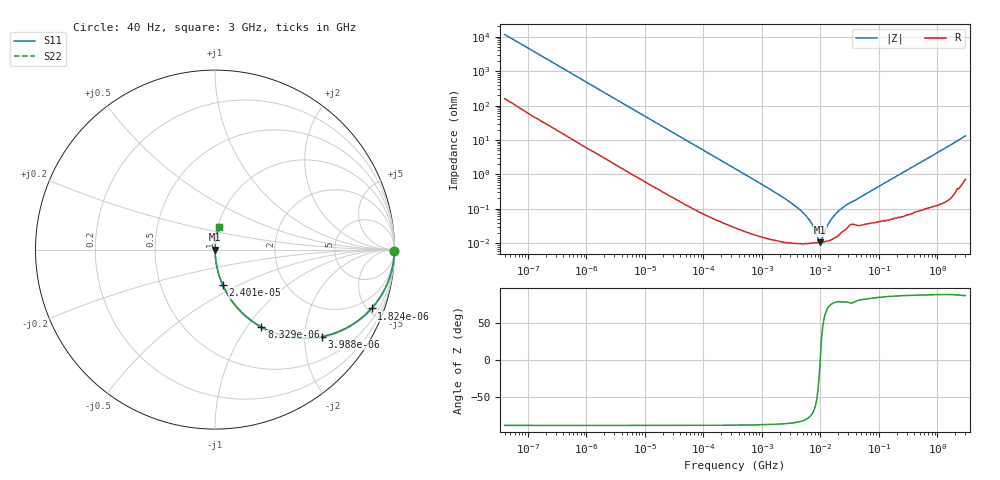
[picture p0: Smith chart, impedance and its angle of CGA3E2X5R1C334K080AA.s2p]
! S-parameter Generated by TDK Corporation
! Copyright(C) 2015 TDK Corporation.
! All Rights Reserved.
! TDK P/N: CGA3E2X5R1C334K080AA (Multilayer Ceramic Chip Capacitors)
! Property: C=330nF
! Size(LxWxT): 1.6x0.8x0.8mm, 0.063x0.031x0.031inches
! Model Type: s2p (Touchstone File Format Version 1.0)
! Frequency: DC=Yes Start=0.00004MHz Stop=3000MHz 396points Log-sweep
! Note: This model was converted from impedance.
! Model Generated on Jun. 23, 2015
! Hash(MD5):
! Port Assignments:
!  1 ---| |--- 2
! Applicable Conditions:
!  Temperature = 25 degC
!  DC Bias Voltage = 0 V
!  Small Signal Operation
! Terms and conditions regarding TDK Simulation Models
! (1)This simulation model is being provided solely for informational purposes. Please refer to the specifications of the products in terms of detailed characteristics of such products.
! (2)In no event shall TDK Corporation of any of its subsidiaries be liable for any loss or damage arising, directly or indirectly,
!  From any information contained in this simulation model, including, but not limited to loss or damages arising from any inaccuracies, omissions or errors in connection with such information.
! (3)Any and all copyrights on this simulation model are owned by TDK Corporation.
!  Duplication or redistribution of this simulation model without prior written permission from TDK Corporation is prohibited.
! (4)This simulation model is subject to any modification or change without any prior notice.
! (5)Neither TDK Corporation nor any of its subsidiaries shall make any warranty, express or implied,
!  Including but not limited to the correctness, implied warranties of merchantability and fitness for a particular purpose with respect to this simulation models.
! (6)The use of this simulation model shall be deemed to have consented to the terms and conditions hereof.
# MHz S MA R 50
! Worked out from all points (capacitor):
!   395 points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, 40 Hz to 3 GHz, reference 50 ohm
!   read as one part in series: C = 340 nF near 41.88 Hz
!   lowest |Z| = 10.7 mohm at 9.97 MHz (marker M1)
!   series resonance near 9.89 MHz, so ESL is about 760 pH
!   S11 on the Smith chart (normalised r, x): 40 Hz: open; 1.824 kHz: 1.07, -5.30; 3.988 kHz: 1.03, -2.44; 8.329 kHz: 1.01, -1.17; 24.01 kHz: 1.01, -0.41; 3 GHz: 1.01, +0.26
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4e-05  0.9998 -0.5  0.008564 88.7  0.008564 88.7  0.9998 -0.5
0.0002520917  0.9979 -3.0  0.05281 86.2  0.05281 86.2  0.9979 -3.0
0.000834128  0.9832 -9.8  0.1707 79.5  0.1707 79.5  0.9832 -9.8
0.001823978  0.9317 -20.6  0.3517 68.7  0.3517 68.7  0.9317 -20.6
0.003988472  0.7684 -39.1  0.6306 50.2  0.6306 50.2  0.7684 -39.1
0.008329251  0.5036 -59.0  0.8577 30.2  0.8577 30.2  0.5036 -59.0
0.01739424  0.2716 -73.5  0.959 15.8  0.959 15.8  0.2716 -73.5
0.02400588  0.2014 -77.7  0.977 11.6  0.977 11.6  0.2014 -77.7
0.0724464  0.06922 -85.3  0.9967 4.0  0.9967 4.0  0.06922 -85.3
0.3464102  0.01478 -88.1  0.9996 0.8  0.9996 0.8  0.01478 -88.1
3.154924  0.00149 -86.0  0.9999 0.1  0.9999 0.1  0.00149 -86.0
4.998775  0.0007861 -83.0  0.9999 0.0  0.9999 0.0  0.0007861 -83.0
7.22376  0.000355 -73.4  0.9999 0.0  0.9999 0.0  0.000355 -73.4
9.521122  0.0001138 -21.5  0.9999 0.0  0.9999 0.0  0.0001138 -21.5
9.969551  0.0001069 4.8  0.9999 -0.0  0.9999 -0.0  0.0001069 4.8
12.54911  0.0002763 65.6  0.9999 -0.0  0.9999 -0.0  0.0002763 65.6
14.40706  0.000427 73.6  0.9999 -0.0  0.9999 -0.0  0.000427 73.6
20.81973  0.0008904 78.6  0.9998 -0.1  0.9998 -0.1  0.0008904 78.6
30.08671  0.00142 77.6  0.9997 -0.1  0.9997 -0.1  0.00142 77.6
150.6385  0.006732 85.5  0.9995 -0.4  0.9995 -0.4  0.006732 85.5
994.0817  0.04251 85.9  0.9978 -2.4  0.9978 -2.4  0.04251 85.9
3000  0.1302 79.4  0.9844 -7.5  0.9844 -7.5  0.1302 79.4
